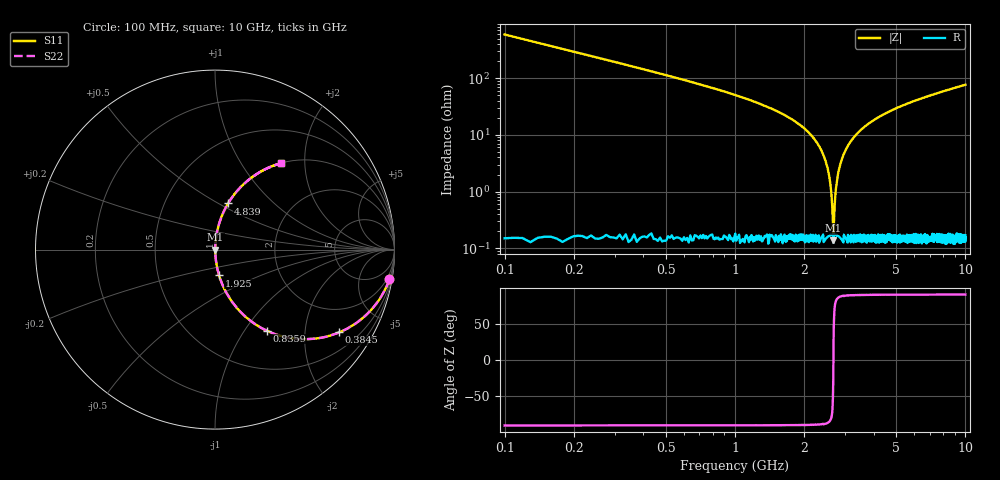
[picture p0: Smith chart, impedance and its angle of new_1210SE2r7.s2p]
!	AVX	Thin	Film	Operation	Date:	April 2007
!	Description:	Accu-P®	"Series,"	Thin	"Film,"	"SMD,"	RF	Capacitor
!	Part	Number:	12101J2R7ABT
!	100	MHz	-	6.05	GHz
!	Serial	Measurements
#	MHZ	S	MA	R	50
!	S11	S21	S12	S22
!	dB	Phase	dB	Phase	dB	Phase	dB	Phase
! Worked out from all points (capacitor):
!   1010 points, 100 MHz to 10 GHz, reference 50 ohm
!   read as one part in series: C = 2.7 pF near 149.1 MHz
!   lowest |Z| = 138 mohm at 2.671 GHz (marker M1)
!   series resonance near 2.674 GHz, so ESL is about 1.3 nH
!   S11 on the Smith chart (normalised r, x): 100 MHz: 1, -12; 384.5 MHz: 1.00, -3.00; 835.9 MHz: 1.00, -1.27; 1.925 GHz: 1.00, -0.30; 4.839 GHz: 1.00, +0.55; 10 GHz: 1.00, +1.53
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100  0.986 -9.6  0.167 80.3  0.167 80.3  0.986 -9.6
237.364  0.926 -22.1  0.376 67.9  0.376 67.9  0.926 -22.1
384.539  0.832 -33.7  0.554 56.3  0.554 56.3  0.832 -33.7
835.877  0.536 -57.4  0.843 32.4  0.843 32.4  0.536 -57.4
1758.176  0.187 -78.8  0.981 10.8  0.981 10.8  0.187 -78.8
1924.975  0.146 -81.0  0.988 8.4  0.988 8.4  0.146 -81.0
2248.761  0.076 -84.5  0.996 4.4  0.996 4.4  0.076 -84.5
2454.807  0.038 -85.6  0.998 2.2  0.998 2.2  0.038 -85.6
2562.735  0.019 -84.4  0.998 1.1  0.998 1.1  0.019 -84.4
2641.229  0.00567 -74.4  0.998 0.3  0.998 0.3  0.00567 -74.4
2670.664  0.00161 -21.5  0.999 0.0  0.999 0.0  0.00161 -21.5
2709.911  0.00602 75.3  0.998 -0.3  0.998 -0.3  0.00602 75.3
2749.158  0.012 82.3  0.998 -0.7  0.998 -0.7  0.012 82.3
2788.404  0.018 84.3  0.998 -1.1  0.998 -1.1  0.018 84.3
2896.333  0.035 85.5  0.998 -2.0  0.998 -2.0  0.035 85.5
3112.19  0.067 84.9  0.996 -3.8  0.996 -3.8  0.067 84.9
3406.541  0.107 83.1  0.993 -6.1  0.993 -6.1  0.107 83.1
4839.049  0.267 74.2  0.962 -15.5  0.962 -15.5  0.267 74.2
5054.906  0.287 73.0  0.957 -16.7  0.957 -16.7  0.287 73.0
6703.271  0.421 64.9  0.906 -24.9  0.906 -24.9  0.421 64.9
8351.635  0.525 58.2  0.85 -31.7  0.85 -31.7  0.525 58.2
10000  0.607 52.5  0.793 -37.4  0.793 -37.4  0.607 52.5
